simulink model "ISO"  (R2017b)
settings: Solver=FixedStepDiscrete  StartTime=0.0  StopTime=10.0  FixedStep=0.01  RelTol=1e-3  EnableMultiTasking=on
undefined symbols (not defined in the file): ASWTYPE_FALSE, ASWTYPE_TRUE, CcISO_CTCOnlineDelayTime_ms, CcISO_FirLvlDebTime_ms, CcISO_FirLvlResChrg_kohm, CcISO_FirLvlResNotChrg_kohm, CcISO_InitDiagDebMaxTi_ms, CcISO_InitDiagDebTi_ms, CcISO_IsoDefaultValue_kohm, CcISO_IsoFastDectectInsVal_kohm, CcISO_IsoFastDetectCnf_MS, CcISO_IsoFastDetectVal_kohm, CcISO_IsoMeasDelayTime_ms, CcISO_ISONegVoltDebTime_ms, CcISO_ISONegVoltFliterDiff_V, CcISO_ISOPackVoltMax_V, CcISO_ISOPackVoltMin_V, CcISO_ISOResCnfFltCnt_NUMB, CcISO_ISOResCnfFltVal_kohm, CcISO_ISOResCnfWarnCnt_NUMB, CcISO_ISOResCnfWarnVal_kohm, CcISO_ISOResNvmMin_kohm, CcISO_ISOResValueinit_kohm, CcISO_IsoResVldVal_NUMB, CcISO_ISOSlopeDelayTime_ms, CcISO_ISOSlopeFilterVal_NUMB, CcISO_NegStMeasFiltTi_ms, CcISO_NegVoltHighRat_pct, CcISO_NegVoltLowRat_pct, CcISO_NorLvlResChrg_kohm, CcISO_NorLvlResNotChrg_kohm, CcISO_PosStMeasFiltTi_ms, CcISO_ResSelfCheckDebTime_ms, CcISO_SedLvlDebTime_ms, CcISO_SedLvlResChrg_kohm, CcISO_SedLvlResNotChrg_kohm, Enum_CTCCtrCtlConnMode, Enum_CTCCtrCtlState, Enum_ISOHVIsoFltLevel, Enum_ISOHVIsoMeasState, Enum_LDPCC2St, Enum_MSMBMUState, ISO_CONST0_NUMB, ISO_CONST1000_NUMB, ISO_CONST1_NUMB, ISO_RESRB1_OHM, ISO_RESRB2_OHM, ISO_RESRS1_OHM, ISO_RESRS2_OHM, ISO_RUNTIME_MS
libraries: AIWAYS_Powertrain_BMS_lib x49
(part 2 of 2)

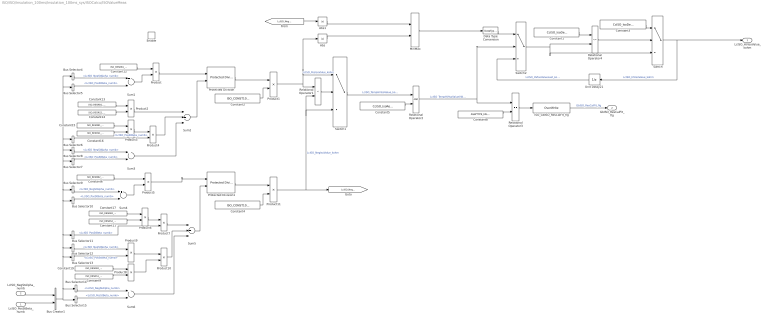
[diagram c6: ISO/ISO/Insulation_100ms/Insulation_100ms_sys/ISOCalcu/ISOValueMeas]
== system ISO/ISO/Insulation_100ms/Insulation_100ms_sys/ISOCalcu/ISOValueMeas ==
  LcISO_PosStBeta_numb : Inport
  LcISO_NegStAlpha_numb : Inport  Port=2
  Enable : EnablePort
  Abs : Abs
  Abs1 : Abs
  Bus Creator1 : BusCreator  Inputs=2
  Bus Selector{5..7,10..11,13,15} (7 alike) : BusSelector  OutputSignals=LcISO_PosStBeta_numb
  Bus Selector{4,8..9,12,14} (5 alike) : BusSelector  OutputSignals=LcISO_NegStAlpha_numb
  Constant1 : Constant  Value=CcISO_IsoDefaultValue_kohm
  Constant11 : Constant  Value=ISO_RESRS2_OHM
  Constant12 : Constant  Value=ISO_RESRB1_OHM
  Constant13 : Constant  Value=ISO_RESRB1_OHM
  Constant14 : Constant  Value=ISO_RESRS2_OHM
  Constant15 : Constant  Value=ISO_RESRB1_OHM
  Constant16 : Constant  Value=ISO_RESRS1_OHM
  Constant17 : Constant  Value=ISO_RESRB2_OHM
  Constant19 : Constant  Value=ISO_RESRB2_OHM
  Constant2 : Constant  Value=ISO_CONST1000_NUMB
  Constant3 : Constant  Value=CcISO_IsoDefaultValue_kohm
  Constant4 : Constant  Value=ISO_CONST1000_NUMB
  Constant5 : Constant  Value=CcISO_IsoResVldVal_NUMB
  Constant6 : Constant  Value=ISO_RESRB2_OHM
  Constant8 : Constant  Value=ASWTYPE_FALSE
  Constant9 : Constant  Value=ISO_RESRS1_OHM
  Data Type Conversion : DataTypeConversion
  ISO_GbISO_ResCalFlt_flg : AIWAYS_Powertrain_BMS_lib/Signals/OverWrite  OverWrite_Value=CbISO_ResCalFltOvr_flg  OverWrite_flag=CbISO_ResCalFltOvrSwt_flg
  MinMax : MinMax  Inputs=2  OutDataTypeStr=Inherit: Inherit via back propagation  RndMeth=Zero
  Product{,4..5,7,9..10} (6 alike) : Product  OutDataTypeStr=Inherit: Inherit via back propagation
  Product{1..3,6,8,11} (6 alike) : Product  Inputs=*/  OutDataTypeStr=Inherit: Inherit via back propagation
  Protected Division : AIWAYS_Powertrain_BMS_lib/Arithmetic Operators/Protected Division
  Protected Division1 : AIWAYS_Powertrain_BMS_lib/Arithmetic Operators/Protected Division
  Relational Operator1 : RelationalOperator  Operator=<  OutDataTypeStr=boolean
  Relational Operator2 : RelationalOperator  OutDataTypeStr=boolean
  Relational Operator3 : RelationalOperator  Operator===  OutDataTypeStr=boolean
  Relational Operator4 : RelationalOperator  Operator=<=  OutDataTypeStr=boolean
  Sum{1,3..4,6} (4 alike) : Sum  Inputs=+-  OutDataTypeStr=Inherit: Inherit via back propagation  RndMeth=Zero
  Sum2 : Sum  Inputs=++-  OutDataTypeStr=Inherit: Inherit via back propagation  RndMeth=Zero
  Sum5 : Sum  Inputs=++-  OutDataTypeStr=Inherit: Inherit via back propagation  RndMeth=Zero
  Switch : Switch  Criteria=u2 ~= 0
  Switch1 : Switch  Criteria=u2 ~= 0  Threshold=1  RndMeth=Zero
  Switch2 : Switch  Criteria=u2 ~= 0
  Unit Delay21 : UnitDelay  InitialCondition=CcISO_ISOResValueinit_kohm  SampleTime=-1  StateName=StateName
  LcISO_HVIsoValue_kohm : Outport
  GbISO_ResCalFlt_flg : Outport  Port=2
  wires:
  Constant3/1 -> Switch/1
  Switch1/1 -> Relational Operator2/1  "LcISO_TempHVIsoValue_kohm"
  Constant1/1 -> Relational Operator4/1
  LcISO_NegStAlpha_numb/1 -> Bus Creator1/1
  LcISO_PosStBeta_numb/1 -> Bus Creator1/2
  Sum1/1 -> Product/2
  Constant12/1 -> Product/1
  Constant13/1 -> Product2/1
  Constant14/1 -> Product2/2
  Constant15/1 -> Product3/1
  Constant16/1 -> Product3/2
  Product3/1 -> Product4/1
  Bus Selector6/1 -> Product4/2  "<LcISO_PosStBeta_numb>"
  Sum3/1 -> Sum2/3
  Product2/1 -> Sum2/1
  Product4/1 -> Sum2/2
  Bus Selector12/1 -> Product9/1  "<LcISO_NegStAlpha_numb>"
  Bus Selector13/1 -> Product9/2  "<LcISO_PosStBeta_numb>"
  Bus Selector11/1 -> Product7/2  "<LcISO_PosStBeta_numb>"
  Constant6/1 -> Product5/1
  Sum4/1 -> Product5/2
  Constant17/1 -> Product6/1
  Constant11/1 -> Product6/2
  Product6/1 -> Product7/1
  Product8/1 -> Product10/2
  Constant9/1 -> Product8/2
  Constant19/1 -> Product8/1
  Product9/1 -> Product10/1
  Product7/1 -> Sum5/1
  Product10/1 -> Sum5/2
  Sum6/1 -> Sum5/3
  Bus Creator1/1 -> Bus Selector6/1, Bus Selector4/1, Bus Selector5/1, Bus Selector8/1, Bus Selector7/1, Bus Selector9/1, Bus Selector10/1, Bus Selector11/1, Bus Selector12/1, Bus Selector13/1, Bus Selector14/1, Bus Selector15/1
  Relational Operator1/1 -> Switch1/2
  Constant2/1 -> Product1/2
  Constant4/1 -> Product11/2
  Relational Operator2/1 -> Relational Operator3/1, Switch2/2  "LcISO_TempHVIsoValueVld_flag"
  Constant5/1 -> Relational Operator2/2
  Constant8/1 -> Relational Operator3/2
  Relational Operator3/1 -> ISO_GbISO_ResCalFlt_flg/1
  ISO_GbISO_ResCalFlt_flg/1 -> GbISO_ResCalFlt_flg/1  "GbISO_ResCalFlt_flg"
  Product1/1 -> Switch1/1, Abs/1, Relational Operator1/1  "LcISO_PosIsoValue_kohm"
  Product11/1 -> [LcISO_NegIsoValue_kohm], Relational Operator1/2, Switch1/3  "LcISO_NegIsoValue_kohm"
  Switch/1 -> Unit Delay21/1, LcISO_HVIsoValue_kohm/1  "LcISO_HVIsoValue_kohm"
  Bus Selector5/1 -> Sum1/2  "<LcISO_PosStBeta_numb>"
  Bus Selector4/1 -> Sum1/1  "<LcISO_NegStAlpha_numb>"
  Bus Selector8/1 -> Sum3/1  "<LcISO_NegStAlpha_numb>"
  Bus Selector7/1 -> Sum3/2  "<LcISO_PosStBeta_numb>"
  Bus Selector9/1 -> Sum4/1  "<LcISO_NegStAlpha_numb>"
  Bus Selector10/1 -> Sum4/2  "<LcISO_PosStBeta_numb>"
  Bus Selector14/1 -> Sum6/1  "<LcISO_NegStAlpha_numb>"
  Bus Selector15/1 -> Sum6/2  "<LcISO_PosStBeta_numb>"
  Product/1 -> Protected Division/1
  Protected Division/1 -> Product1/1
  Sum2/1 -> Protected Division/2
  Protected Division1/1 -> Product11/1
  Product5/1 -> Protected Division1/1
  Sum5/1 -> Protected Division1/2
  Unit Delay21/1 -> Switch2/3  "LcISO_HVIsoValueLast_kohm"
  Data Type Conversion/1 -> Switch2/1
  Relational Operator4/1 -> Switch/2
  Switch2/1 -> Switch/3, Relational Operator4/2
  [LcISO_NegIsoValue_kohm] -> Abs1/1
  Abs1/1 -> MinMax/1
  Abs/1 -> MinMax/2
  MinMax/1 -> Data Type Conversion/1

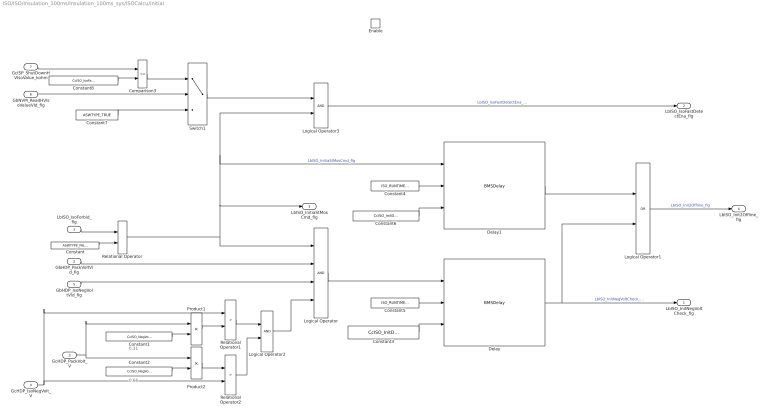
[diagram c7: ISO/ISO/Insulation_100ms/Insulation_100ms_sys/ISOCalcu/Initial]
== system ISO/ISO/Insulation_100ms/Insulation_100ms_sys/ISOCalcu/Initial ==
  note: 0.31
  note: 0.66
  LbISO_IsoForbid_flg : Inport
  GbHDP_PackVoltVld_flg : Inport  Port=2
  GcHDP_PackVolt_V : Inport  Port=3
  GcHDP_IsoNegVolt_V : Inport  Port=4
  GbHDP_IsoNegVoltVld_flg : Inport  Port=5
  GbNVM_ReadHVIsoValueVld_flg : Inport  Port=6
  GcISP_ShutDownHVIsoValue_kohm : Inport  Port=7
  Enable : EnablePort  StatesWhenEnabling=reset
  Comparison3 : RelationalOperator  Operator=<=  OutDataTypeStr=boolean
  Constant : Constant  Value=ASWTYPE_FALSE
  Constant1 : Constant  Value=CcISO_NegVoltLowRat_pct
  Constant2 : Constant  Value=CcISO_NegVoltHighRat_pct
  Constant3 : Constant  Value=CcISO_InitDiagDebTi_ms
  Constant4 : Constant  Value=ISO_RUNTIME_MS
  Constant5 : Constant  Value=ISO_RUNTIME_MS
  Constant6 : Constant  Value=CcISO_InitDiagDebMaxTi_ms
  Constant7 : Constant  Value=ASWTYPE_TRUE
  Constant8 : Constant  Value=CcISO_IsoFastDetectVal_kohm
  Delay : AIWAYS_Powertrain_BMS_lib/Debounce & Delay/BMSDelay
  Delay1 : AIWAYS_Powertrain_BMS_lib/Debounce & Delay/BMSDelay
  Logical Operator : Logic  Inputs=4  AllPortsSameDT=off  OutDataTypeStr=boolean
  Logical Operator1 : Logic  Operator=OR  AllPortsSameDT=off  OutDataTypeStr=boolean
  Logical Operator2 : Logic  AllPortsSameDT=off  OutDataTypeStr=boolean
  Logical Operator3 : Logic  AllPortsSameDT=off  OutDataTypeStr=boolean
  Product1 : Product  Inputs=**  OutDataTypeStr=Inherit: Inherit via back propagation
  Product2 : Product  Inputs=**  OutDataTypeStr=Inherit: Inherit via back propagation
  Relational Operator : RelationalOperator  Operator===  OutDataTypeStr=boolean
  Relational Operator1 : RelationalOperator  Operator=>  OutDataTypeStr=boolean
  Relational Operator2 : RelationalOperator  Operator=>  OutDataTypeStr=boolean
  Switch1 : Switch  Criteria=u2 ~= 0
  LbISO_InitNegVoltCheck_flg : Outport
  LbISO_IsoFastDetectEna_flg : Outport  Port=2
  LbISO_InitiaStMosCmd_flg : Outport  Port=3
  LbISO_Init2Offline_flg : Outport  Port=4
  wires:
  Relational Operator/1 -> Logical Operator3/2, Delay1/1, LbISO_InitiaStMosCmd_flg/1, Logical Operator/1  "LbISO_InitiaStMosCmd_flg"
  Constant/1 -> Relational Operator/2
  LbISO_IsoForbid_flg/1 -> Relational Operator/1
  Logical Operator/1 -> Delay/1
  Constant5/1 -> Delay/2
  Constant3/1 -> Delay/3
  Delay/1 -> LbISO_InitNegVoltCheck_flg/1, Logical Operator1/2  "LbISO_InitNegVoltCheck_flg"
  Constant4/1 -> Delay1/2
  Constant6/1 -> Delay1/3
  Delay1/1 -> Logical Operator1/1
  Logical Operator1/1 -> LbISO_Init2Offline_flg/1  "LbISO_Init2Offline_flg"
  Constant1/1 -> Product1/2
  Product1/1 -> Relational Operator1/2
  GcHDP_PackVolt_V/1 -> Product1/1, Product2/1
  GcHDP_IsoNegVolt_V/1 -> Relational Operator1/1, Relational Operator2/2
  Constant2/1 -> Product2/2
  Product2/1 -> Relational Operator2/1
  Relational Operator1/1 -> Logical Operator2/1
  Relational Operator2/1 -> Logical Operator2/2
  Logical Operator2/1 -> Logical Operator/4
  GbHDP_PackVoltVld_flg/1 -> Logical Operator/2
  GbHDP_IsoNegVoltVld_flg/1 -> Logical Operator/3
  Constant7/1 -> Switch1/3
  GcISP_ShutDownHVIsoValue_kohm/1 -> Comparison3/1
  Switch1/1 -> Logical Operator3/1
  GbNVM_ReadHVIsoValueVld_flg/1 -> Switch1/2
  Constant8/1 -> Comparison3/2
  Comparison3/1 -> Switch1/1
  Logical Operator3/1 -> LbISO_IsoFastDetectEna_flg/1  "LbISO_IsoFastDetectEna_flg"

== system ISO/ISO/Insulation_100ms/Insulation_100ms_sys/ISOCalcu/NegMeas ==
  LbISO_IsoForbid_flg : Inport
  GcHDP_IsoNegVolt_V : Inport  Port=2
  GcHDP_PackVolt_V : Inport  Port=3
  Enable : EnablePort  StatesWhenEnabling=reset
  NegLossPassFiter : Subsystem
  NegMeas2Offline : Subsystem
  LcISO_NegStAlpha_numb : Outport
  LbISO_NegMeas2VauleCalcu_flg : Outport  Port=2
  LbISO_NegMeas2Offline_flg : Outport  Port=3
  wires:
  NegMeas2Offline/1(LbISO_NegMeas2Offline_flg) -> LbISO_NegMeas2Offline_flg/1
  LbISO_IsoForbid_flg/1 -> NegMeas2Offline/1(LbISO_IsoForbid_flg)
  NegLossPassFiter/2(LbISO_NegMeas2VauleCalcu_flg) -> LbISO_NegMeas2VauleCalcu_flg/1
  GcHDP_IsoNegVolt_V/1 -> NegLossPassFiter/1(GcHDP_IsoNegVolt_V)
  GcHDP_PackVolt_V/1 -> NegLossPassFiter/2(GcHDP_PackVolt_V)
  NegLossPassFiter/1(LcISO_NegStAlpha_numb) -> LcISO_NegStAlpha_numb/1

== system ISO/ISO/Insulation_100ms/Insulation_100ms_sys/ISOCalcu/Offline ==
  LbISO_IsoForbid_flg : Inport
  Enable : EnablePort  StatesWhenEnabling=reset
  Constant : Constant  Value=ASWTYPE_FALSE
  Relational Operator : RelationalOperator  Operator===  OutDataTypeStr=boolean
  LbISO_Offline2PosMeas_flg : Outport
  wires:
  LbISO_IsoForbid_flg/1 -> Relational Operator/1
  Constant/1 -> Relational Operator/2
  Relational Operator/1 -> LbISO_Offline2PosMeas_flg/1  "LbISO_Offline2PosMeas_flg"

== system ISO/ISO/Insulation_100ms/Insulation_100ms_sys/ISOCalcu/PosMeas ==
  LbISO_IsoForbid_flg : Inport
  GcHDP_IsoNegVolt_V : Inport  Port=2
  GcHDP_PackVolt_V : Inport  Port=3
  Enable : EnablePort  StatesWhenEnabling=reset
  NegLossPassFiter : Subsystem
  PosMeas2Offline : Subsystem
  LbISO_PosMeas2NegMeas_flg : Outport
  LbISO_PosMeas2Offline_flg : Outport  Port=2
  LcISO_PosStBeta_numb : Outport  Port=3
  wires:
  NegLossPassFiter/2(LbISO_PosMeas2NegMeas_flg) -> LbISO_PosMeas2NegMeas_flg/1
  LbISO_IsoForbid_flg/1 -> PosMeas2Offline/1(LbISO_IsoForbid_flg)
  PosMeas2Offline/1(LbISO_PosMeas2Offline_flg) -> LbISO_PosMeas2Offline_flg/1
  GcHDP_IsoNegVolt_V/1 -> NegLossPassFiter/1(GcHDP_IsoNegVolt_V)
  NegLossPassFiter/1(LcISO_PosStBeta_numb) -> LcISO_PosStBeta_numb/1
  GcHDP_PackVolt_V/1 -> NegLossPassFiter/2(GcHDP_PackVolt_V)

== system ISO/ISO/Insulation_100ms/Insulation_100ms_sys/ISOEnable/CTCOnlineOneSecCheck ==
  GeCTC_CtrCtlState_enum : Inport
  Constant3 : Constant  Value=Enum_CTCCtrCtlState.Enum_CTCCtrCtlState_Online
  Constant6 : Constant  Value=ISO_RUNTIME_MS
  Constant7 : Constant  Value=CcISO_CTCOnlineDelayTime_ms
  Constant9 : Constant  Value=ASWTYPE_FALSE
  Delay : AIWAYS_Powertrain_BMS_lib/Debounce & Delay/BMSDelay
  Logical Operator : Logic  AllPortsSameDT=off  OutDataTypeStr=boolean
  Relational Operator : RelationalOperator  Operator===  OutDataTypeStr=boolean
  Relational Operator3 : RelationalOperator  Operator===  OutDataTypeStr=boolean
  LbISO_CTCOnlineTimeReach_flg : Outport
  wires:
  Constant7/1 -> Delay/3
  Constant6/1 -> Delay/2
  Constant3/1 -> Relational Operator3/2
  GeCTC_CtrCtlState_enum/1 -> Relational Operator3/1
  Relational Operator3/1 -> Logical Operator/2, Delay/1
  Delay/1 -> Relational Operator/1
  Logical Operator/1 -> LbISO_CTCOnlineTimeReach_flg/1  "LbISO_CTCOnlineTimeReach_flg"
  Constant9/1 -> Relational Operator/2
  Relational Operator/1 -> Logical Operator/1

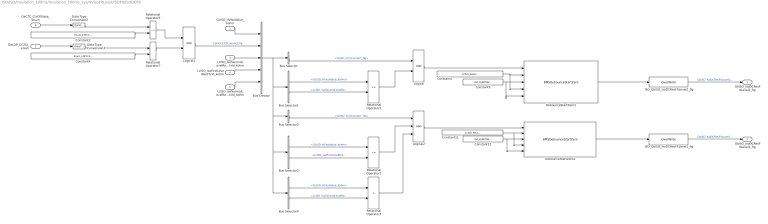
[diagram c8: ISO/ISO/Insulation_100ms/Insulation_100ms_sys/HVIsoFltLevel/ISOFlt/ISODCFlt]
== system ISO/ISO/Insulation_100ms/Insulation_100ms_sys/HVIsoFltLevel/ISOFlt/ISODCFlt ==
  GcISO_HVIsoValue_kohm : Inport
  GeLDP_CC2St_enum : Inport  Port=2
  LcISO_IsoSecondLevelResThrld_kohm : Inport  Port=3
  LcISO_IsoFirstLevelResThrld_kohm : Inport  Port=4
  LcISO_IsoNormalLevelResThrld_kohm : Inport  Port=5
  GeCTC_CtrCtlState_enum : Inport  Port=6
  Bus Creator : BusCreator  Inputs=5
  Bus Selector : BusSelector  OutputSignals=LbISO_CC2Connect_flg
  Bus Selector1 : BusSelector  OutputSignals=GcISO_HVIsoValue_kohm,LcISO_IsoSecondLevelResThrld_kohm
  Bus Selector2 : BusSelector  OutputSignals=GcISO_HVIsoValue_kohm,LcISO_IsoFirstLevelResThrld_kohm
  Bus Selector3 : BusSelector  OutputSignals=LbISO_CC2Connect_flg
  Bus Selector4 : BusSelector  OutputSignals=GcISO_HVIsoValue_kohm,LcISO_IsoSecondLevelResThrld_kohm
  Constant11 : Constant  Value=CcISO_FirLvlDebTime_ms
  Constant12 : Constant  Value=ISO_RUNTIME_MS
  Constant2 : Constant  Value=Enum_CTCCtrCtlState.Enum_CTCCtrCtlState_Offline
  Constant4 : Constant  Value=Enum_LDPCC2St.Enum_LDPCC2St_Connect
  Constant5 : Constant  Value=CcISO_SedLvlDebTime_ms
  Constant6 : Constant  Value=ISO_RUNTIME_MS
  Data Type Conversion2 : DataTypeConversion
  Data Type Conversion3 : DataTypeConversion
  DebounceStartZero1 : AIWAYS_Powertrain_BMS_lib/Debounce & Delay/BMSDebounceStartZero
  DebounceStartZero2 : AIWAYS_Powertrain_BMS_lib/Debounce & Delay/BMSDebounceStartZero
  ISO_GbISO_IsoDCResFltLevel1_flg : AIWAYS_Powertrain_BMS_lib/Signals/OverWrite  OverWrite_Value=CbISO_IsoDCResFltLevel1Ovr_flg  OverWrite_flag=CbISO_IsoDCResFltLevel1OvrSwt_flg
  ISO_GbISO_IsoDCResFltLevel2_flg : AIWAYS_Powertrain_BMS_lib/Signals/OverWrite  OverWrite_Value=CbISO_IsoDCResFltLevel2Ovr_flg  OverWrite_flag=CbISO_IsoDCResFltLevel2OvrSwt_flg
  Logical : Logic  OutDataTypeStr=boolean
  Logical1 : Logic  OutDataTypeStr=boolean
  Logical2 : Logic  Inputs=3  OutDataTypeStr=boolean
  Relational Operator1 : RelationalOperator  Operator=<=  OutDataTypeStr=boolean
  Relational Operator2 : RelationalOperator  Operator=<=  OutDataTypeStr=boolean
  Relational Operator3 : RelationalOperator  Operator=>  OutDataTypeStr=boolean
  Relational Operator5 : RelationalOperator  Operator=~=  OutDataTypeStr=boolean
  Relational Operator7 : RelationalOperator  Operator===  OutDataTypeStr=boolean
  GbISO_IsoDCResFltLevel2_flg : Outport
  GbISO_IsoDCResFltLevel1_flg : Outport  Port=2
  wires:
  ISO_GbISO_IsoDCResFltLevel2_flg/1 -> GbISO_IsoDCResFltLevel2_flg/1  "GbISO_IsoDCResFltLevel2_flg"
  ISO_GbISO_IsoDCResFltLevel1_flg/1 -> GbISO_IsoDCResFltLevel1_flg/1  "GbISO_IsoDCResFltLevel1_flg"
  LcISO_IsoFirstLevelResThrld_kohm/1 -> Bus Creator/4
  Constant12/1 -> DebounceStartZero2/5, DebounceStartZero2/3
  Logical1/1 -> Bus Creator/2  "LbISO_CC2Connect_flg"
  GcISO_HVIsoValue_kohm/1 -> Bus Creator/1
  LcISO_IsoSecondLevelResThrld_kohm/1 -> Bus Creator/3
  LcISO_IsoNormalLevelResThrld_kohm/1 -> Bus Creator/5
  Constant11/1 -> DebounceStartZero2/2, DebounceStartZero2/4
  Bus Selector1/1 -> Relational Operator1/1  "<GcISO_HVIsoValue_kohm>"
  Bus Selector3/1 -> Logical2/1  "<LbISO_CC2Connect_flg>"
  Bus Selector1/2 -> Relational Operator1/2  "<LcISO_IsoSecondLevelResThrld_kohm>"
  Relational Operator2/1 -> Logical2/2
  Constant5/1 -> DebounceStartZero1/2, DebounceStartZero1/4
  Bus Selector2/2 -> Relational Operator2/2  "<LcISO_IsoFirstLevelResThrld_kohm>"
  Logical/1 -> DebounceStartZero1/1
  Constant6/1 -> DebounceStartZero1/3, DebounceStartZero1/5
  Bus Selector2/1 -> Relational Operator2/1  "<GcISO_HVIsoValue_kohm>"
  Bus Creator/1 -> Bus Selector4/1, Bus Selector2/1, Bus Selector3/1, Bus Selector1/1, Bus Selector/1
  Logical2/1 -> DebounceStartZero2/1
  Bus Selector/1 -> Logical/1  "<LbISO_CC2Connect_flg>"
  Relational Operator1/1 -> Logical/2
  Bus Selector4/1 -> Relational Operator3/1  "<GcISO_HVIsoValue_kohm>"
  Bus Selector4/2 -> Relational Operator3/2  "<LcISO_IsoSecondLevelResThrld_kohm>"
  Relational Operator3/1 -> Logical2/3
  GeLDP_CC2St_enum/1 -> Data Type Conversion3/1
  Constant4/1 -> Relational Operator7/2
  Data Type Conversion3/1 -> Relational Operator7/1
  Relational Operator7/1 -> Logical1/2
  DebounceStartZero1/1 -> ISO_GbISO_IsoDCResFltLevel2_flg/1
  DebounceStartZero2/1 -> ISO_GbISO_IsoDCResFltLevel1_flg/1
  Constant2/1 -> Relational Operator5/2
  GeCTC_CtrCtlState_enum/1 -> Data Type Conversion2/1
  Data Type Conversion2/1 -> Relational Operator5/1
  Relational Operator5/1 -> Logical1/1

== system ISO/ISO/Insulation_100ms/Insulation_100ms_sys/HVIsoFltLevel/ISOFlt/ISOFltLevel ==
  GbISO_IsoResFltLevel2_flg : Inport
  GbISO_IsoResFltLevel1_flg : Inport  Port=2
  GbISO_IsoHVoffResFltLevel2_flg : Inport  Port=3
  GbISO_IsoHVoffResFltLevel1_flg : Inport  Port=4
  GbISO_IsoDCResFltLevel2_flg : Inport  Port=5
  GbISO_IsoDCResFltLevel1_flg : Inport  Port=6
  Bus Creator : BusCreator  Inputs=6
  Bus Selector : BusSelector  OutputSignals=GbISO_IsoResFltLevel2_flg,GbISO_IsoHVoffResFltLevel2_flg,GbISO_IsoDCResFltLevel2_flg
  Bus Selector1 : BusSelector  OutputSignals=GbISO_IsoResFltLevel1_flg,GbISO_IsoHVoffResFltLevel1_flg,GbISO_IsoDCResFltLevel1_flg
  Constant13 : Constant  Value=Enum_ISOHVIsoFltLevel.Enum_ISOHVIsoFltLevel_FltLevel2
  Constant17 : Constant  Value=Enum_ISOHVIsoFltLevel.Enum_ISOHVIsoFltLevel_Default
  Constant8 : Constant  Value=Enum_ISOHVIsoFltLevel.Enum_ISOHVIsoFltLevel_FltLevel3
  Data Type Conversion4 : DataTypeConversion
  ISO_GeISO_ResFltLvl_enum : AIWAYS_Powertrain_BMS_lib/Signals/OverWrite  OverWrite_Value=CeISO_ResFltLvlOvr_enum  OverWrite_flag=CbISO_ResFltLvlOvrSwt_flg
  Logical1 : Logic  Operator=OR  Inputs=3  OutDataTypeStr=boolean
  Logical2 : Logic  Operator=OR  Inputs=3  OutDataTypeStr=boolean
  Switch1 : Switch  Criteria=u2 ~= 0  OutDataTypeStr=Inherit: Inherit via back propagation
  Switch2 : Switch  Criteria=u2 ~= 0  OutDataTypeStr=Inherit: Inherit via back propagation
  GeISO_ResFltLvl_enum : Outport
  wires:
  Logical2/1 -> Switch2/2
  Constant13/1 -> Switch2/1
  Constant8/1 -> Switch1/1
  Switch2/1 -> Switch1/3
  Logical1/1 -> Switch1/2
  Constant17/1 -> Switch2/3
  ISO_GeISO_ResFltLvl_enum/1 -> GeISO_ResFltLvl_enum/1  "GeISO_ResFltLvl_enum"
  Switch1/1 -> Data Type Conversion4/1
  Data Type Conversion4/1 -> ISO_GeISO_ResFltLvl_enum/1
  GbISO_IsoResFltLevel2_flg/1 -> Bus Creator/1
  GbISO_IsoHVoffResFltLevel2_flg/1 -> Bus Creator/2
  GbISO_IsoDCResFltLevel2_flg/1 -> Bus Creator/3
  GbISO_IsoResFltLevel1_flg/1 -> Bus Creator/4
  GbISO_IsoHVoffResFltLevel1_flg/1 -> Bus Creator/5
  GbISO_IsoDCResFltLevel1_flg/1 -> Bus Creator/6
  Bus Creator/1 -> Bus Selector1/1, Bus Selector/1
  Bus Selector/1 -> Logical1/1  "<GbISO_IsoResFltLevel2_flg>"
  Bus Selector/2 -> Logical1/2  "<GbISO_IsoHVoffResFltLevel2_flg>"
  Bus Selector/3 -> Logical1/3  "<GbISO_IsoDCResFltLevel2_flg>"
  Bus Selector1/1 -> Logical2/1  "<GbISO_IsoResFltLevel1_flg>"
  Bus Selector1/2 -> Logical2/2  "<GbISO_IsoHVoffResFltLevel1_flg>"
  Bus Selector1/3 -> Logical2/3  "<GbISO_IsoDCResFltLevel1_flg>"

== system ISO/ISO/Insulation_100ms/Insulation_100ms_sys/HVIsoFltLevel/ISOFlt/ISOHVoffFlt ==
  GcISO_HVIsoValue_kohm : Inport
  GeCTC_CtrCtlState_enum : Inport  Port=2
  LcISO_IsoSecondLevelResThrld_kohm : Inport  Port=3
  LcISO_IsoFirstLevelResThrld_kohm : Inport  Port=4
  LcISO_IsoNormalLevelResThrld_kohm : Inport  Port=5
  Bus Creator : BusCreator  Inputs=5
  Bus Selector : BusSelector  OutputSignals=LbISO_CtrCtlHVoff_flg
  Bus Selector1 : BusSelector  OutputSignals=GcISO_HVIsoValue_kohm,LcISO_IsoSecondLevelResThrld_kohm
  Bus Selector2 : BusSelector  OutputSignals=GcISO_HVIsoValue_kohm,LcISO_IsoFirstLevelResThrld_kohm
  Bus Selector3 : BusSelector  OutputSignals=LbISO_CtrCtlHVoff_flg
  Bus Selector4 : BusSelector  OutputSignals=GcISO_HVIsoValue_kohm,LcISO_IsoSecondLevelResThrld_kohm
  Constant11 : Constant  Value=CcISO_FirLvlDebTime_ms
  Constant12 : Constant  Value=ISO_RUNTIME_MS
  Constant3 : Constant  Value=Enum_CTCCtrCtlState.Enum_CTCCtrCtlState_Offline
  Constant5 : Constant  Value=CcISO_SedLvlDebTime_ms
  Constant6 : Constant  Value=ISO_RUNTIME_MS
  Data Type Conversion1 : DataTypeConversion
  DebounceStartZero1 : AIWAYS_Powertrain_BMS_lib/Debounce & Delay/BMSDebounceStartZero
  DebounceStartZero2 : AIWAYS_Powertrain_BMS_lib/Debounce & Delay/BMSDebounceStartZero
  ISO_GbISO_IsoHVoffResFltLevel1_flg : AIWAYS_Powertrain_BMS_lib/Signals/OverWrite  OverWrite_Value=CbISO_IsoHVoffResFltLevel1Ovr_flg  OverWrite_flag=CbISO_IsoHVoffResFltLevel1OvrSwt_flg
  ISO_GbISO_IsoHVoffResFltLevel2_flg : AIWAYS_Powertrain_BMS_lib/Signals/OverWrite  OverWrite_Value=CbISO_IsoHVoffResFltLevel2Ovr_flg  OverWrite_flag=CbISO_IsoHVoffResFltLevel2OvrSwt_flg
  Logical : Logic  OutDataTypeStr=boolean
  Logical1 : Logic  Operator=OR  OutDataTypeStr=boolean
  Logical2 : Logic  Inputs=3  OutDataTypeStr=boolean
  Relational Operator1 : RelationalOperator  Operator=<=  OutDataTypeStr=boolean
  Relational Operator11 : RelationalOperator  Operator===  OutDataTypeStr=boolean
  Relational Operator2 : RelationalOperator  Operator=<=  OutDataTypeStr=boolean
  Relational Operator4 : RelationalOperator  Operator=>  OutDataTypeStr=boolean
  Unit Delay21 : UnitDelay  InitialCondition=ASWTYPE_FALSE  SampleTime=-1  StateName=StateName
  GbISO_IsoHVoffResFltLevel2_flg : Outport
  GbISO_IsoHVoffResFltLevel1_flg : Outport  Port=2
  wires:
  Constant12/1 -> DebounceStartZero2/5, DebounceStartZero2/3
  Constant11/1 -> DebounceStartZero2/2, DebounceStartZero2/4
  ISO_GbISO_IsoHVoffResFltLevel1_flg/1 -> GbISO_IsoHVoffResFltLevel1_flg/1  "GbISO_IsoHVoffResFltLevel1_flg"
  ISO_GbISO_IsoHVoffResFltLevel2_flg/1 -> GbISO_IsoHVoffResFltLevel2_flg/1  "GbISO_IsoHVoffResFltLevel2_flg"
  Constant6/1 -> DebounceStartZero1/3, DebounceStartZero1/5
  Constant5/1 -> DebounceStartZero1/2, DebounceStartZero1/4
  DebounceStartZero2/1 -> ISO_GbISO_IsoHVoffResFltLevel1_flg/1
  Unit Delay21/1 -> Logical1/2
  DebounceStartZero1/1 -> Logical1/1
  Logical1/1 -> ISO_GbISO_IsoHVoffResFltLevel2_flg/1, Unit Delay21/1
  GcISO_HVIsoValue_kohm/1 -> Bus Creator/1
  Relational Operator11/1 -> Bus Creator/2  "LbISO_CtrCtlHVoff_flg"
  LcISO_IsoSecondLevelResThrld_kohm/1 -> Bus Creator/3
  LcISO_IsoFirstLevelResThrld_kohm/1 -> Bus Creator/4
  LcISO_IsoNormalLevelResThrld_kohm/1 -> Bus Creator/5
  Bus Creator/1 -> Bus Selector4/1, Bus Selector2/1, Bus Selector3/1, Bus Selector1/1, Bus Selector/1
  Bus Selector1/1 -> Relational Operator1/1  "<GcISO_HVIsoValue_kohm>"
  Bus Selector1/2 -> Relational Operator1/2  "<LcISO_IsoSecondLevelResThrld_kohm>"
  Bus Selector2/1 -> Relational Operator2/1  "<GcISO_HVIsoValue_kohm>"
  Bus Selector2/2 -> Relational Operator2/2  "<LcISO_IsoFirstLevelResThrld_kohm>"
  Data Type Conversion1/1 -> Relational Operator11/1
  Constant3/1 -> Relational Operator11/2
  GeCTC_CtrCtlState_enum/1 -> Data Type Conversion1/1
  Bus Selector/1 -> Logical/1  "<LbISO_CtrCtlHVoff_flg>"
  Relational Operator1/1 -> Logical/2
  Logical/1 -> DebounceStartZero1/1
  Logical2/1 -> DebounceStartZero2/1
  Relational Operator2/1 -> Logical2/2
  Bus Selector3/1 -> Logical2/1  "<LbISO_CtrCtlHVoff_flg>"
  Relational Operator4/1 -> Logical2/3
  Bus Selector4/2 -> Relational Operator4/2  "<LcISO_IsoSecondLevelResThrld_kohm>"
  Bus Selector4/1 -> Relational Operator4/1  "<GcISO_HVIsoValue_kohm>"

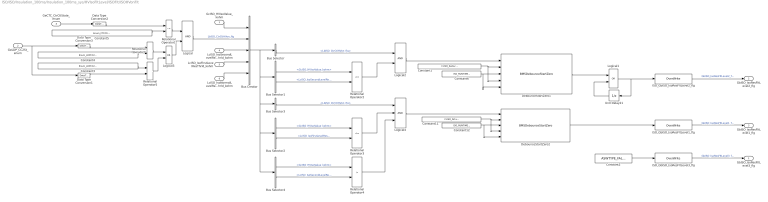
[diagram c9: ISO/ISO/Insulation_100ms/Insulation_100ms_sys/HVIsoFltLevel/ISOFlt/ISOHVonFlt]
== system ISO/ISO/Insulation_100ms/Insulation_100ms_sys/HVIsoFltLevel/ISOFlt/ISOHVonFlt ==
  GcISO_HVIsoValue_kohm : Inport
  GeLDP_CC2St_enum : Inport  Port=2
  GeCTC_CtrCtlState_enum : Inport  Port=3
  LcISO_IsoSecondLevelResThrld_kohm : Inport  Port=4
  LcISO_IsoFirstLevelResThrld_kohm : Inport  Port=5
  LcISO_IsoNormalLevelResThrld_kohm : Inport  Port=6
  Bus Creator : BusCreator  Inputs=5
  Bus Selector : BusSelector  OutputSignals=LbISO_CtrCtlHVon_flg
  Bus Selector1 : BusSelector  OutputSignals=GcISO_HVIsoValue_kohm,LcISO_IsoSecondLevelResThrld_kohm
  Bus Selector2 : BusSelector  OutputSignals=GcISO_HVIsoValue_kohm,LcISO_IsoFirstLevelResThrld_kohm
  Bus Selector3 : BusSelector  OutputSignals=LbISO_CtrCtlHVon_flg
  Bus Selector4 : BusSelector  OutputSignals=GcISO_HVIsoValue_kohm,LcISO_IsoSecondLevelResThrld_kohm
  Constant1 : Constant  Value=CcISO_SedLvlDebTime_ms
  Constant11 : Constant  Value=CcISO_FirLvlDebTime_ms
  Constant12 : Constant  Value=ISO_RUNTIME_MS
  Constant2 : Constant  Value=ASWTYPE_FALSE
  Constant3 : Constant  Value=Enum_LDPCC2St.Enum_LDPCC2St_Fault
  Constant4 : Constant  Value=Enum_LDPCC2St.Enum_LDPCC2St_Unconnect
  Constant5 : Constant  Value=Enum_CTCCtrCtlState.Enum_CTCCtrCtlState_Offline
  Constant6 : Constant  Value=ISO_RUNTIME_MS
  Data Type Conversion1 : DataTypeConversion
  Data Type Conversion2 : DataTypeConversion
  Data Type Conversion3 : DataTypeConversion
  DebounceStartZero1 : AIWAYS_Powertrain_BMS_lib/Debounce & Delay/BMSDebounceStartZero
  DebounceStartZero2 : AIWAYS_Powertrain_BMS_lib/Debounce & Delay/BMSDebounceStartZero
  ISO_GbISO_IsoResFltLevel1_flg : AIWAYS_Powertrain_BMS_lib/Signals/OverWrite  OverWrite_Value=CbISO_IsoResFltLevel1Ovr_flg  OverWrite_flag=CbISO_IsoResFltLevel1OvrSwt_flg
  ISO_GbISO_IsoResFltLevel2_flg : AIWAYS_Powertrain_BMS_lib/Signals/OverWrite  OverWrite_Value=CbISO_IsoResFltLevel2Ovr_flg  OverWrite_flag=CbISO_IsoResFltLevel2OvrSwt_flg
  ISO_GbISO_IsoResFltLevel3_flg : AIWAYS_Powertrain_BMS_lib/Signals/OverWrite  OverWrite_Value=CbISO_IsoResFltLevel3Ovr_flg  OverWrite_flag=CbISO_IsoResFltLevel3OvrSwt_flg
  Logical : Logic  OutDataTypeStr=boolean
  Logical1 : Logic  Operator=OR  OutDataTypeStr=boolean
  Logical2 : Logic  OutDataTypeStr=boolean
  Logical3 : Logic  Operator=OR  OutDataTypeStr=boolean
  Logical4 : Logic  Inputs=3  OutDataTypeStr=boolean
  Relational Operator1 : RelationalOperator  Operator=~=  OutDataTypeStr=boolean
  Relational Operator2 : RelationalOperator  Operator=<=  OutDataTypeStr=boolean
  Relational Operator3 : RelationalOperator  Operator=<=  OutDataTypeStr=boolean
  Relational Operator4 : RelationalOperator  Operator=>  OutDataTypeStr=boolean
  Relational Operator5 : RelationalOperator  Operator===  OutDataTypeStr=boolean
  Relational Operator7 : RelationalOperator  Operator===  OutDataTypeStr=boolean
  Unit Delay21 : UnitDelay  InitialCondition=ASWTYPE_FALSE  SampleTime=-1  StateName=StateName
  GbISO_IsoResFltLevel3_flg : Outport
  GbISO_IsoResFltLevel2_flg : Outport  Port=2
  GbISO_IsoResFltLevel1_flg : Outport  Port=3
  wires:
  Logical1/1 -> ISO_GbISO_IsoResFltLevel2_flg/1, Unit Delay21/1
  DebounceStartZero1/1 -> Logical1/1
  Unit Delay21/1 -> Logical1/2
  Constant2/1 -> ISO_GbISO_IsoResFltLevel3_flg/1
  ISO_GbISO_IsoResFltLevel3_flg/1 -> GbISO_IsoResFltLevel3_flg/1  "GbISO_IsoResFltLevel3_flg"
  ISO_GbISO_IsoResFltLevel2_flg/1 -> GbISO_IsoResFltLevel2_flg/1  "GbISO_IsoResFltLevel2_flg"
  ISO_GbISO_IsoResFltLevel1_flg/1 -> GbISO_IsoResFltLevel1_flg/1  "GbISO_IsoResFltLevel1_flg"
  LcISO_IsoFirstLevelResThrld_kohm/1 -> Bus Creator/4
  GeCTC_CtrCtlState_enum/1 -> Data Type Conversion2/1
  GcISO_HVIsoValue_kohm/1 -> Bus Creator/1
  LcISO_IsoSecondLevelResThrld_kohm/1 -> Bus Creator/3
  LcISO_IsoNormalLevelResThrld_kohm/1 -> Bus Creator/5
  Data Type Conversion2/1 -> Relational Operator1/1
  Constant5/1 -> Relational Operator1/2
  Constant4/1 -> Relational Operator7/2
  Data Type Conversion3/1 -> Relational Operator7/1
  GeLDP_CC2St_enum/1 -> Data Type Conversion1/1, Data Type Conversion3/1
  Relational Operator1/1 -> Logical/1
  Relational Operator7/1 -> Logical3/1
  Logical/1 -> Bus Creator/2  "LbISO_CtrCtlHVon_flg"
  Constant12/1 -> DebounceStartZero2/5, DebounceStartZero2/3
  Constant11/1 -> DebounceStartZero2/2, DebounceStartZero2/4
  Bus Selector1/1 -> Relational Operator2/1  "<GcISO_HVIsoValue_kohm>"
  Bus Selector3/1 -> Logical4/1  "<LbISO_CtrCtlHVon_flg>"
  Bus Selector1/2 -> Relational Operator2/2  "<LcISO_IsoSecondLevelResThrld_kohm>"
  Relational Operator3/1 -> Logical4/2
  Constant1/1 -> DebounceStartZero1/2, DebounceStartZero1/4
  Bus Selector2/2 -> Relational Operator3/2  "<LcISO_IsoFirstLevelResThrld_kohm>"
  Logical4/1 -> DebounceStartZero2/1
  Bus Creator/1 -> Bus Selector/1, Bus Selector2/1, Bus Selector4/1, Bus Selector3/1, Bus Selector1/1
  Logical2/1 -> DebounceStartZero1/1
  Constant6/1 -> DebounceStartZero1/3, DebounceStartZero1/5
  Bus Selector2/1 -> Relational Operator3/1  "<GcISO_HVIsoValue_kohm>"
  Relational Operator2/1 -> Logical2/2
  Bus Selector/1 -> Logical2/1  "<LbISO_CtrCtlHVon_flg>"
  DebounceStartZero2/1 -> ISO_GbISO_IsoResFltLevel1_flg/1
  Bus Selector4/2 -> Relational Operator4/2  "<LcISO_IsoSecondLevelResThrld_kohm>"
  Bus Selector4/1 -> Relational Operator4/1  "<GcISO_HVIsoValue_kohm>"
  Relational Operator4/1 -> Logical4/3
  Logical3/1 -> Logical/2
  Constant3/1 -> Relational Operator5/1
  Relational Operator5/1 -> Logical3/2
  Data Type Conversion1/1 -> Relational Operator5/2

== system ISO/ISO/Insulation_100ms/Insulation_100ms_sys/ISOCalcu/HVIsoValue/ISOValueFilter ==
  note: 750k≥R＞250k
  note: R≤250k
  LcISO_HVIsoValue_kohm : Inport
  Enable : EnablePort
  Comparison : RelationalOperator  Operator=>  OutDataTypeStr=boolean
  Comparison1 : RelationalOperator  Operator=>  OutDataTypeStr=boolean
  Constant1 : Constant  Value=CcISO_ISOResCnfFltCnt_NUMB
  Constant2 : Constant  Value=CcISO_ISOResCnfFltVal_kohm
  Constant3 : Constant  Value=CcISO_ISOResCnfWarnCnt_NUMB
  Constant4 : Constant  Value=CcISO_ISOResCnfWarnVal_kohm
  Logical : Logic  OutDataTypeStr=boolean
  Logical1 : Logic  Operator=NOT  OutDataTypeStr=boolean
  Logical2 : Logic  Operator=NOT  OutDataTypeStr=boolean
  Logical3 : Logic  Operator=OR  Inputs=3  OutDataTypeStr=boolean
  Switch3 : Switch  Criteria=u2 ~= 0
  Turn On Delay Sample : AIWAYS_Powertrain_BMS_lib/Delay Blocks/Turn On Delay Sample
  Turn On Delay Sample1 : AIWAYS_Powertrain_BMS_lib/Delay Blocks/Turn On Delay Sample
  Unit Delay3 : UnitDelay  SampleTime=-1  StateName=StateName
  LcISO_HVIsoValueFilter_kohm : Outport
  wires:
  Constant2/1 -> Comparison/2
  Comparison/1 -> Logical/1, Logical1/1
  Switch3/1 -> Unit Delay3/1, LcISO_HVIsoValueFilter_kohm/1  "LcISO_HVIsoValueFilter_kohm"
  Logical1/1 -> Turn On Delay Sample/2
  Constant1/1 -> Turn On Delay Sample/1
  Unit Delay3/1 -> Switch3/3
  Constant4/1 -> Comparison1/2
  Logical2/1 -> Logical/2
  Comparison1/1 -> Logical2/1, Logical3/2  "LbISO_HVIsoValueFilterFlg2_flg"
  Turn On Delay Sample1/1 -> Logical3/3  "LbISO_HVIsoValueFilterFlg3_flg"
  Turn On Delay Sample/1 -> Logical3/1  "LbISO_HVIsoValueFilterFlg1_flg"
  Logical3/1 -> Switch3/2
  Logical/1 -> Turn On Delay Sample1/2
  Constant3/1 -> Turn On Delay Sample1/1
  LcISO_HVIsoValue_kohm/1 -> Switch3/1, Comparison1/1, Comparison/1

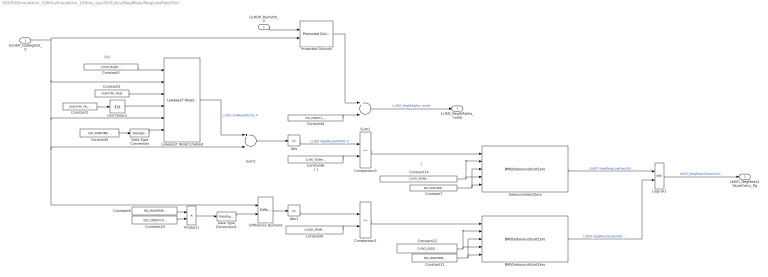
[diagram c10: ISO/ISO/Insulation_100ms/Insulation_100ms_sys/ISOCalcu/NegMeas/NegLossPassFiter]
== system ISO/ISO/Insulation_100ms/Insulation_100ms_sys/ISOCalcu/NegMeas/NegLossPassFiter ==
  note: 500
  note: 1.3
  note: 1
  GcHDP_IsoNegVolt_V : Inport
  GcHDP_PackVolt_V : Inport  Port=2
  Abs : Abs
  Abs1 : Abs
  BMSDebounceStartZero : AIWAYS_Powertrain_BMS_lib/Debounce & Delay/BMSDebounceStartZero
  Comparison1 : RelationalOperator  Operator=<=  OutDataTypeStr=boolean
  Comparison3 : RelationalOperator  Operator=<=  OutDataTypeStr=boolean
  Constant1 : Constant  Value=ASWTYPE_FALSE
  Constant10 : Constant  Value=ISO_CONST1000_NUMB
  Constant{5,7..8,11} (4 alike) : Constant  Value=ISO_RUNTIME_MS
  Constant12 : Constant  Value=CcISO_ISOSlopeDelayTime_ms
  Constant14 : Constant  Value=CcISO_ISONegVoltDebTime_ms
  Constant2 : Constant  Value=ASWTYPE_TRUE
  Constant3 : Constant  Value=CcISO_NegStMeasFiltTi_ms
  Constant4 : Constant  Value=ISO_CONST1_NUMB
  Constant6 : Constant  Value=CcISO_ISONegVoltFliterDiff_V
  Constant9 : Constant  Value=CcISO_ISOSlopeFilterVal_NUMB
  Data Type Conversion : DataTypeConversion  OutDataTypeStr=uint16
  Data Type Conversion1 : DataTypeConversion
  DebounceStartZero : AIWAYS_Powertrain_BMS_lib/Debounce & Delay/BMSDebounceStartZero
  Difference Quotient : AIWAYS_Powertrain_BMS_lib/Obsolete Blocks/Difference Quotient
  Logical1 : Logic  OutDataTypeStr=boolean
  LowpassT Reset Enabled : AIWAYS_Powertrain_BMS_lib/Filters & Averages/LowpassT Reset Enabled
  Product1 : Product  Inputs=*/  OutDataTypeStr=Inherit: Inherit via back propagation
  Protected Division : AIWAYS_Powertrain_BMS_lib/Arithmetic Operators/Protected Division
  Sum1 : Sum  Inputs=+-  RndMeth=Zero
  Sum2 : Sum  Inputs=+-  RndMeth=Zero
  Unit Delay1 : UnitDelay  InitialCondition=ASWTYPE_TRUE  SampleTime=-1  StateName=StateName
  LcISO_NegStAlpha_numb : Outport
  LbISO_NegMeas2VauleCalcu_flg : Outport  Port=2
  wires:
  Constant5/1 -> Data Type Conversion/1
  Constant2/1 -> LowpassT Reset Enabled/3
  Constant1/1 -> Unit Delay1/1
  GcHDP_IsoNegVolt_V/1 -> LowpassT Reset Enabled/2, Difference Quotient/1, Sum2/2, LowpassT Reset Enabled/5, Protected Division/2
  Constant3/1 -> LowpassT Reset Enabled/1
  Unit Delay1/1 -> LowpassT Reset Enabled/4
  Sum1/1 -> LcISO_NegStAlpha_numb/1  "LcISO_NegStAlpha_numb"
  Data Type Conversion/1 -> LowpassT Reset Enabled/6
  Protected Division/1 -> Sum1/1
  Constant4/1 -> Sum1/2
  LowpassT Reset Enabled/1 -> Sum2/1  "LcISO_IsoNegVoltUn2_V"
  GcHDP_PackVolt_V/1 -> Protected Division/1
  Sum2/1 -> Abs/1
  Constant6/1 -> Comparison3/2
  Abs/1 -> Comparison3/1  "LcISO_NegMeasVoltDiff_V"
  Constant14/1 -> DebounceStartZero/2, DebounceStartZero/4
  Constant7/1 -> DebounceStartZero/3, DebounceStartZero/5
  Comparison3/1 -> DebounceStartZero/1
  Logical1/1 -> LbISO_NegMeas2VauleCalcu_flg/1  "LbISO_NegMeas2VauleCalcu_flg"
  DebounceStartZero/1 -> Logical1/1  "LbISO_NegMeasLowPassVld_flg"
  Data Type Conversion1/1 -> Difference Quotient/2
  Abs1/1 -> Comparison1/1
  Product1/1 -> Data Type Conversion1/1
  Constant12/1 -> BMSDebounceStartZero/2, BMSDebounceStartZero/4
  Comparison1/1 -> BMSDebounceStartZero/1
  Difference Quotient/1 -> Abs1/1
  Constant8/1 -> Product1/1
  Constant11/1 -> BMSDebounceStartZero/3, BMSDebounceStartZero/5
  Constant9/1 -> Comparison1/2
  BMSDebounceStartZero/1 -> Logical1/2  "LbISO_NegMeasSlopeVld2_flg"
  Constant10/1 -> Product1/2

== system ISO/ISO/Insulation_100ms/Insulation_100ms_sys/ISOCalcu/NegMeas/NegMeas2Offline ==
  LbISO_IsoForbid_flg : Inport
  Constant1 : Constant  Value=ASWTYPE_TRUE
  Constant2 : Constant  Value=ASWTYPE_TRUE
  Constant5 : Constant  Value=ISO_RUNTIME_MS
  Constant6 : Constant  Value=CcISO_IsoMeasDelayTime_ms
  Delay : AIWAYS_Powertrain_BMS_lib/Debounce & Delay/BMSDelay
  Logical1 : Logic  Operator=OR  OutDataTypeStr=boolean
  Relational Operator2 : RelationalOperator  Operator===  OutDataTypeStr=boolean
  LbISO_NegMeas2Offline_flg : Outport
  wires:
  Constant2/1 -> Relational Operator2/2
  LbISO_IsoForbid_flg/1 -> Relational Operator2/1
  Logical1/1 -> LbISO_NegMeas2Offline_flg/1  "LbISO_NegMeas2Offline_flg"
  Constant6/1 -> Delay/3
  Constant5/1 -> Delay/2
  Constant1/1 -> Delay/1
  Delay/1 -> Logical1/2
  Relational Operator2/1 -> Logical1/1

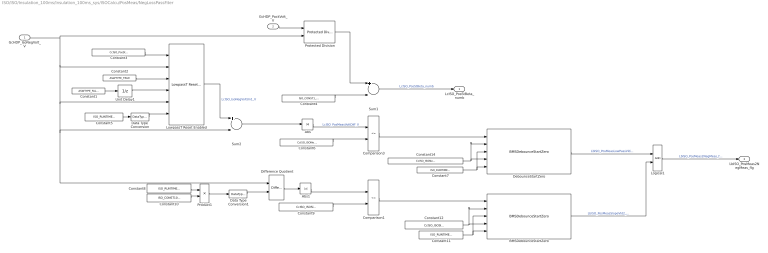
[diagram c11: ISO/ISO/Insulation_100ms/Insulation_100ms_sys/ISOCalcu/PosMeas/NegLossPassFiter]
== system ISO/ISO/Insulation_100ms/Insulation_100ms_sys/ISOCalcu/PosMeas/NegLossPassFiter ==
  GcHDP_IsoNegVolt_V : Inport
  GcHDP_PackVolt_V : Inport  Port=2
  Abs : Abs
  Abs1 : Abs
  BMSDebounceStartZero : AIWAYS_Powertrain_BMS_lib/Debounce & Delay/BMSDebounceStartZero
  Comparison1 : RelationalOperator  Operator=<=  OutDataTypeStr=boolean
  Comparison3 : RelationalOperator  Operator=<=  OutDataTypeStr=boolean
  Constant1 : Constant  Value=ASWTYPE_FALSE
  Constant10 : Constant  Value=ISO_CONST1000_NUMB
  Constant{5,7..8,11} (4 alike) : Constant  Value=ISO_RUNTIME_MS
  Constant12 : Constant  Value=CcISO_ISOSlopeDelayTime_ms
  Constant14 : Constant  Value=CcISO_ISONegVoltDebTime_ms
  Constant2 : Constant  Value=ASWTYPE_TRUE
  Constant3 : Constant  Value=CcISO_PosStMeasFiltTi_ms
  Constant4 : Constant  Value=ISO_CONST1_NUMB
  Constant6 : Constant  Value=CcISO_ISONegVoltFliterDiff_V
  Constant9 : Constant  Value=CcISO_ISOSlopeFilterVal_NUMB
  Data Type Conversion : DataTypeConversion  OutDataTypeStr=uint16
  Data Type Conversion1 : DataTypeConversion
  DebounceStartZero : AIWAYS_Powertrain_BMS_lib/Debounce & Delay/BMSDebounceStartZero
  Difference Quotient : AIWAYS_Powertrain_BMS_lib/Obsolete Blocks/Difference Quotient
  Logical1 : Logic  OutDataTypeStr=boolean
  LowpassT Reset Enabled : AIWAYS_Powertrain_BMS_lib/Filters & Averages/LowpassT Reset Enabled
  Product1 : Product  Inputs=*/  OutDataTypeStr=Inherit: Inherit via back propagation
  Protected Division : AIWAYS_Powertrain_BMS_lib/Arithmetic Operators/Protected Division
  Sum1 : Sum  Inputs=+-  RndMeth=Zero
  Sum2 : Sum  Inputs=+-  RndMeth=Zero
  Unit Delay1 : UnitDelay  InitialCondition=ASWTYPE_TRUE  SampleTime=-1  StateName=StateName
  LcISO_PosStBeta_numb : Outport
  LbISO_PosMeas2NegMeas_flg : Outport  Port=2
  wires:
  Constant2/1 -> LowpassT Reset Enabled/3
  Constant1/1 -> Unit Delay1/1
  Unit Delay1/1 -> LowpassT Reset Enabled/4
  Constant5/1 -> Data Type Conversion/1
  Constant3/1 -> LowpassT Reset Enabled/1
  Sum1/1 -> LcISO_PosStBeta_numb/1  "LcISO_PosStBeta_numb"
  Data Type Conversion/1 -> LowpassT Reset Enabled/6
  Protected Division/1 -> Sum1/1
  Constant4/1 -> Sum1/2
  LowpassT Reset Enabled/1 -> Sum2/1  "LcISO_IsoNegVoltUn1_V"
  GcHDP_PackVolt_V/1 -> Protected Division/1
  Sum2/1 -> Abs/1
  Abs/1 -> Comparison3/1  "LcISO_PosMeasVoltDiff_V"
  Constant6/1 -> Comparison3/2
  Constant7/1 -> DebounceStartZero/3, DebounceStartZero/5
  Constant14/1 -> DebounceStartZero/2, DebounceStartZero/4
  Comparison3/1 -> DebounceStartZero/1
  Logical1/1 -> LbISO_PosMeas2NegMeas_flg/1  "LbISO_PosMeas2NegMeas_flg"
  DebounceStartZero/1 -> Logical1/1  "LbISO_PosMeasLowPassVld_flg"
  Constant12/1 -> BMSDebounceStartZero/2, BMSDebounceStartZero/4
  Data Type Conversion1/1 -> Difference Quotient/2
  GcHDP_IsoNegVolt_V/1 -> LowpassT Reset Enabled/5, Sum2/2, Difference Quotient/1, LowpassT Reset Enabled/2, Protected Division/2
  Constant11/1 -> BMSDebounceStartZero/3, BMSDebounceStartZero/5
  Constant8/1 -> Product1/1
  Difference Quotient/1 -> Abs1/1
  Abs1/1 -> Comparison1/1
  Constant9/1 -> Comparison1/2
  Product1/1 -> Data Type Conversion1/1
  BMSDebounceStartZero/1 -> Logical1/2  "LbISO_PosMeasSlopeVld2_flg"
  Constant10/1 -> Product1/2
  Comparison1/1 -> BMSDebounceStartZero/1

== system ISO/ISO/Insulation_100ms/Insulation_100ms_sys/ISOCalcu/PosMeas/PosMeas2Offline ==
  LbISO_IsoForbid_flg : Inport
  Constant1 : Constant  Value=ASWTYPE_TRUE
  Constant2 : Constant  Value=ASWTYPE_TRUE
  Constant5 : Constant  Value=ISO_RUNTIME_MS
  Constant6 : Constant  Value=CcISO_IsoMeasDelayTime_ms
  Delay : AIWAYS_Powertrain_BMS_lib/Debounce & Delay/BMSDelay
  Logical1 : Logic  Operator=OR  OutDataTypeStr=boolean
  Relational Operator2 : RelationalOperator  Operator===  OutDataTypeStr=boolean
  LbISO_PosMeas2Offline_flg : Outport
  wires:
  Logical1/1 -> LbISO_PosMeas2Offline_flg/1  "LbISO_PosMeas2Offline_flg"
  LbISO_IsoForbid_flg/1 -> Relational Operator2/1
  Constant2/1 -> Relational Operator2/2
  Constant1/1 -> Delay/1
  Constant6/1 -> Delay/3
  Delay/1 -> Logical1/2
  Relational Operator2/1 -> Logical1/1
  Constant5/1 -> Delay/2

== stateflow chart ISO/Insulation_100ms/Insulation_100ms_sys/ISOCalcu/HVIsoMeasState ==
  state Initial
    en:
    LeISO_HVIsoMeasState_enum = Enum_ISOHVIsoMeasState.Enum_ISOHVIsoMeasState_Initial;
    GbISO_PosMosCmd_flg = ASWTYPE_FALSE;
    GbISO_NegMosCmd_flg = ASWTYPE_FALSE;
    LcISO_IsoFastDetectCnt_MS = ISO_CONST0_NUMB;
    du:
    LcISO_IsoFastDetectCnt_MS += ISO_RUNTIME_MS;
    ex:
    LcISO_IsoFastDetectCnt_MS = ISO_CONST0_NUMB;
  state FastDetect
    en:
    GbISO_PosMosCmd_flg = LbISO_InitiaStMosCmd_flg;
    GbISO_NegMosCmd_flg = LbISO_InitiaStMosCmd_flg;
    du:
    GbISO_PosMosCmd_flg = LbISO_InitiaStMosCmd_flg;
    GbISO_NegMosCmd_flg = LbISO_InitiaStMosCmd_flg;
  state Offline
    en:
    LeISO_HVIsoMeasState_enum = Enum_ISOHVIsoMeasState.Enum_ISOHVIsoMeasState_Offline;
    GbISO_PosMosCmd_flg = ASWTYPE_FALSE;
    GbISO_NegMosCmd_flg = ASWTYPE_FALSE;
  state PosMeas
    en:
    LeISO_HVIsoMeasState_enum = Enum_ISOHVIsoMeasState.Enum_ISOHVIsoMeasState_PosMeas;
    GbISO_PosMosCmd_flg = ASWTYPE_TRUE;
    GbISO_NegMosCmd_flg = ASWTYPE_FALSE;
    ex:
    GbISO_PosMosCmd_flg = ASWTYPE_FALSE;
    GbISO_NegMosCmd_flg = ASWTYPE_FALSE;
  state NegMeas
    en:
    LeISO_HVIsoMeasState_enum = Enum_ISOHVIsoMeasState.Enum_ISOHVIsoMeasState_NegMeas;
    GbISO_NegMosCmd_flg = ASWTYPE_TRUE;
    GbISO_PosMosCmd_flg = ASWTYPE_FALSE;
    ex:
    GbISO_NegMosCmd_flg = ASWTYPE_FALSE;
    GbISO_PosMosCmd_flg = ASWTYPE_FALSE;
  state VauleMeas
    en:
    LeISO_HVIsoMeasState_enum = Enum_ISOHVIsoMeasState.Enum_ISOHVIsoMeasState_VauleCalcu;
  (default) -> Initial
  Initial -> Offline : [ASWTYPE_TRUE == LbISO_Init2Offline_flg]
  Initial -> Offline : [ASWTYPE_FALSE == LbISO_IsoFastDetectEna_flg &&... LcISO_IsoFastDetectCnt_MS >= CcISO_IsoFastDetectCnf_MS]
  Initial -> FastDetect : [ASWTYPE_TRUE == LbISO_IsoFastDetectEna_flg]
  FastDetect -> Offline : [ASWTYPE_TRUE == LbISO_Init2Offline_flg]
  NegMeas -> Offline : [ASWTYPE_TRUE == LbISO_NegMeas2Offline_flg]
  VauleMeas -> Offline
  PosMeas -> Offline : [ASWTYPE_TRUE ==LbISO_PosMeas2Offline_flg]
  Offline -> PosMeas : [ASWTYPE_TRUE == LbISO_Offline2PosMeas_flg]
  PosMeas -> NegMeas : [ASWTYPE_TRUE == LbISO_PosMeas2NegMeas_flg]
  NegMeas -> VauleMeas : [ASWTYPE_TRUE == LbISO_NegMeas2VauleCalcu_flg]
  data: LbISO_InitNegVoltCheck_flg input; LbISO_IsoFastDetectEna_flg input; LbISO_InitiaStMosCmd_flg input; LbISO_Init2Offline_flg input; LeISO_HVIsoMeasState_enum output; GbISO_PosMosCmd_flg output; GbISO_NegMosCmd_flg output; LbISO_Offline2PosMeas_flg input; LbISO_PosMeas2NegMeas_flg input; LbISO_PosMeas2Offline_flg input; LbISO_NegMeas2VauleCalcu_flg input; ASWTYPE_TRUE parameter; LbISO_NegMeas2Offline_flg input; ASWTYPE_FALSE parameter; CcISO_IsoFastDetectCnf_MS parameter; LcISO_IsoFastDetectCnt_MS local double; ISO_CONST0_NUMB parameter; ISO_RUNTIME_MS parameter
